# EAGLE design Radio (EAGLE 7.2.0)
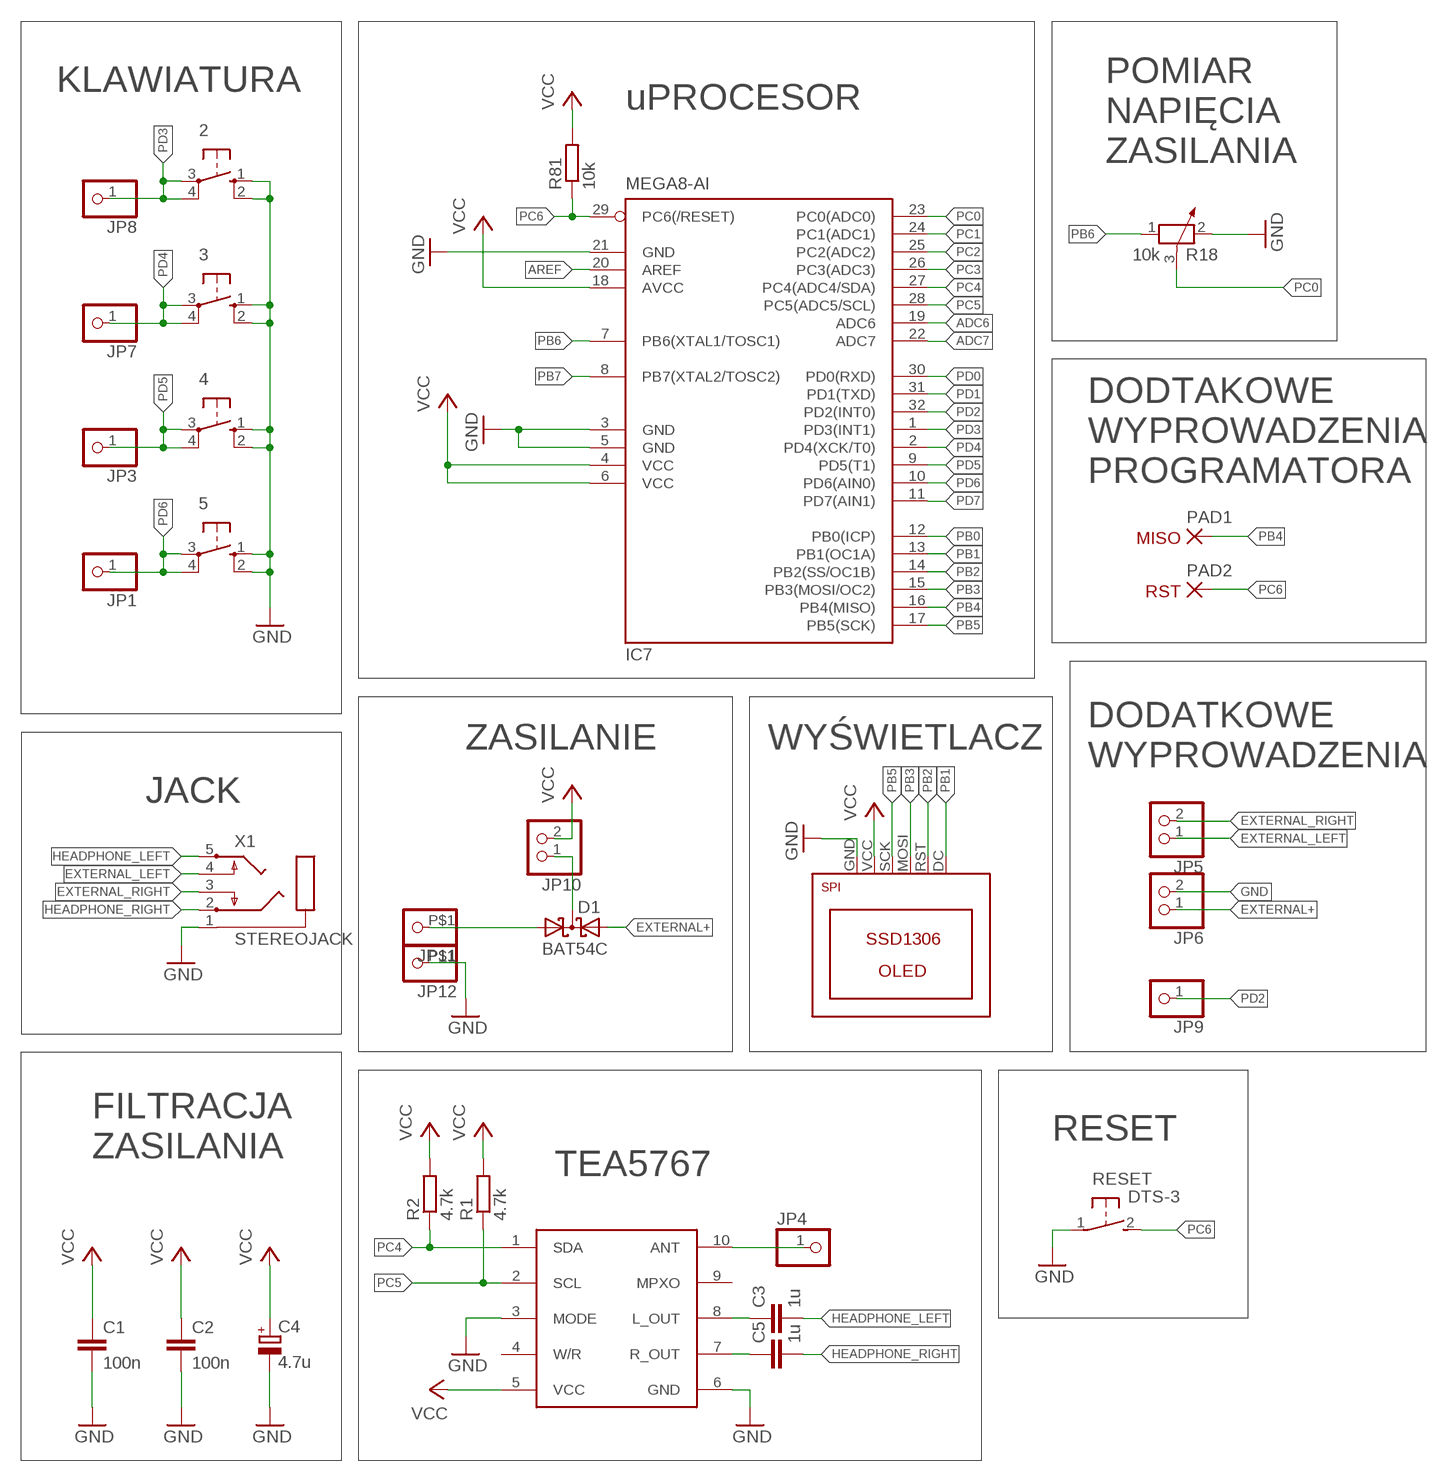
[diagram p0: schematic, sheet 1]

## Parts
2  10-XX  [B3F-10XX]
3  10-XX  [B3F-10XX]
4  10-XX  [B3F-10XX]
5  10-XX  [B3F-10XX]
C1  100n  C-EUC0805  [C0805]
C2  100n  C-EUC0805  [C0805]
C3  1u  C-EUC0805  [C0805]
C4  4.7u  CPOL-EUB/3528-21R  [B/3528-21R]
C5  1u  C-EUC0805  [C0805]
D1  BAT54C  [SOT23]
IC7  MEGA8-AI  [TQFP32-08]
JP1  PINHD-1X01_2.54-90°  [1X01/90]
JP3  PINHD-1X01_2.54-90°  [1X01/90]
JP4  PINHD-1X01_2.54-90°  [1X01/90]
JP5  PINHD-1X02_2.54  [1X02]
JP6  PINHD-1X02_2.54  [1X02]
JP7  PINHD-1X01_2.54-90°  [1X01/90]
JP8  PINHD-1X01_2.54-90°  [1X01/90]
JP9  PINHD-1X01_2.54-90°  [1X01/90]
JP10  PINHD-1X02_2.54  [1X02]
JP11  PINHD-1X01  [1X01_OFFSET]
JP12  PINHD-1X01  [1X01_OFFSET]
PAD1  SMD2  [SMD1,27-2,54]
PAD2  SMD2  [SMD1,27-2,54]
R1  4.7k  R-EU_R0805  [R0805]
R2  4.7k  R-EU_R0805  [R0805]
R18  10k  POTENTIOMETER_  [WH06-2A]
R81  10k  R-EU_R0805  [R0805]
RESET  DTS-3  [DTS-3]
U$1  TEA5767BREAKOUT  [TEA5767MM2]
U$2  SPINEW  [SSD1306_SPI_NO_CS_NO_HOLES]
X1  STEREOJACK  [STX3100]

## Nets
ADC6: IC7.19(ADC6)
ADC7: IC7.22(ADC7)
AREF: IC7.20(AREF)
BATTERY+: D1.1(A1) JP11.P$1
EXTERNAL+: D1.2(A2) JP6.1
EXTERNAL_LEFT: JP5.1 X1.4
EXTERNAL_RIGHT: JP5.2 X1.3
GND: 2.1(S) 2.2(S1) 3.1(S) 3.2(S1) 4.1(S) 4.2(S1) 5.1(S) 5.2(S1) C1.2 C2.2 C4.- IC7.3(GND) IC7.5(GND) IC7.21(GND) JP6.2 JP12.P$1 R18.2 RESET.1 U$1.3(MODE) U$1.6(GND) U$2.GND X1.1
HEADPHONE_LEFT: C3.2 X1.5
HEADPHONE_RIGHT: C5.2 X1.2
N$1: JP4.1 U$1.10(ANT)
N$2: D1.3(CC) JP10.1
N$3: C3.1 U$1.8(L_OUT)
N$4: C5.1 U$1.7(R_OUT)
PB0: IC7.12(PB0(ICP))
PB1: IC7.13(PB1(OC1A)) U$2.DC
PB2: IC7.14(PB2(SS/OC1B)) U$2.RST
PB3: IC7.15(PB3(MOSI/OC2)) U$2.MOSI
PB4: IC7.16(PB4(MISO)) PAD1.1(P)
PB5: IC7.17(PB5(SCK)) U$2.SCK
PB6: IC7.7(PB6(XTAL1/TOSC1)) R18.1
PB7: IC7.8(PB7(XTAL2/TOSC2))
PC0: IC7.23(PC0(ADC0)) R18.3
PC1: IC7.24(PC1(ADC1))
PC2: IC7.25(PC2(ADC2))
PC3: IC7.26(PC3(ADC3))
PC4: IC7.27(PC4(ADC4/SDA)) R2.1 U$1.1(SDA)
PC5: IC7.28(PC5(ADC5/SCL)) R1.1 U$1.2(SCL)
PC6: IC7.29(PC6(/RESET)) PAD2.1(P) R81.1 RESET.2
PD0: IC7.30(PD0(RXD))
PD1: IC7.31(PD1(TXD))
PD2: IC7.32(PD2(INT0)) JP9.1
PD3: 2.3(P) 2.4(P1) IC7.1(PD3(INT1)) JP8.1
PD4: 3.3(P) 3.4(P1) IC7.2(PD4(XCK/T0)) JP7.1
PD5: 4.3(P) 4.4(P1) IC7.9(PD5(T1)) JP3.1
PD6: 5.3(P) 5.4(P1) IC7.10(PD6(AIN0)) JP1.1
PD7: IC7.11(PD7(AIN1))
VCC: C1.1 C2.1 C4.+ IC7.4(VCC) IC7.6(VCC) IC7.18(AVCC) JP10.2 R1.2 R2.2 R81.2 U$1.5(VCC) U$2.VCC
Unconnected: U$1.4(W/R) U$1.9(MPXO)

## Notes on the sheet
- KLAWIATURA
- uPROCESOR
- POMIAR
  NAPIĘCIA
  ZASILANIA
- DODTAKOWE
  WYPROWADZENIA
  PROGRAMATORA
- MISO
- RST
- ZASILANIE | WYŚWIETLACZ
- DODATKOWE
  WYPROWADZENIA
- JACK
- RESET
- FILTRACJA
  ZASILANIA
- TEA5767

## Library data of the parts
2-5 = switch-omron:10-XX: OMRON SWITCH; MPN: B3F-1000; OC_FARNELL: 176432; OC_NEWARK: 36M3542
C1-C3 C5 = rcl:C-EU: CAPACITOR, European symbol
C4 = rcl:CPOL-EU: POLARIZED CAPACITOR, European symbol
D1 = diode:BAT54C: Schottky Diodes Source: Fairchild .. BAT54.pdf
IC7 = atmel:MEGA8: MICROCONTROLLER 8 Kbytes FLASH, 1 kbytes SRAM, 512 bytes EEPROM, USART, 6-channel 10 bit ADC, 2-channel 8 bit ADC Pin compatible with Atmega48, ATMega88, ATMega168 Source: avr.lbr; MPN: ATMEGA8-16AU; OC_FARNELL: 9171371; OC_NEWARK: 73M8863
JP1 JP3 JP4 JP7-JP9 = pinhead_my:PINHD-1X01: PIN HEADER
JP5 JP6 JP10 = pinhead_my:PINHD-1X02: PIN HEADER
JP11 JP12 = pinhead-2:PINHD-1X01: PIN HEADER
PAD1 PAD2 = wirepad:SMD2: SMD PAD
R1 R2 R81 = rcl:R-EU_: RESISTOR, European symbol
R18 = potencjometr:POTENTIOMETER_: Potentiometer
RESET = switch-tact:DTS-3
U$1 = MyParts:TEA5767BREAKOUT
U$2 = ssd1306_breakout_board:SPI
X1 = adafruit:STEREOJACK: MIC/HEADPHONE JACK Stereo jack with two switches. Kycon STX3100, CUI SJ1-3555NG and/or 4UCon 05544

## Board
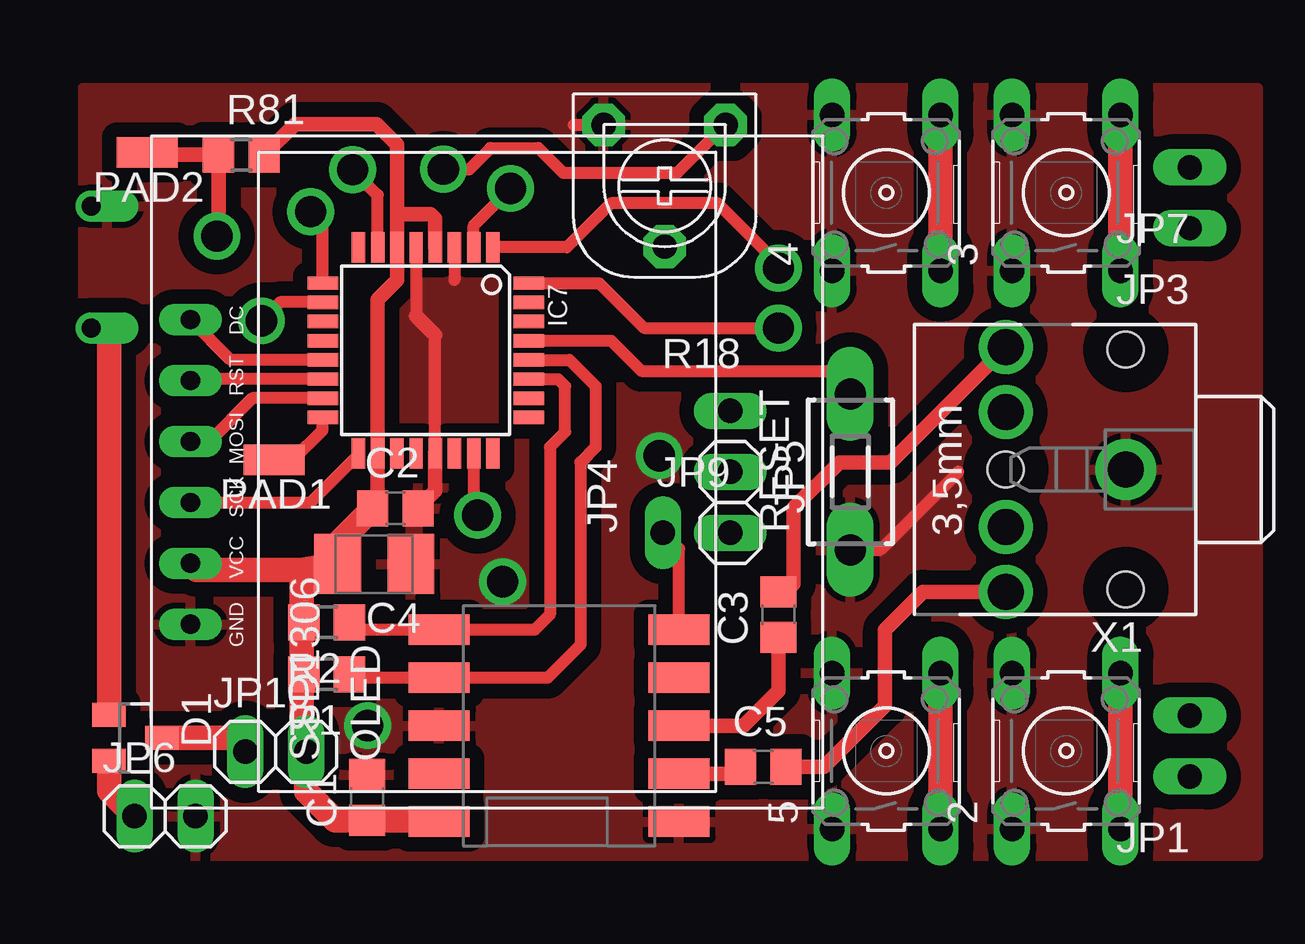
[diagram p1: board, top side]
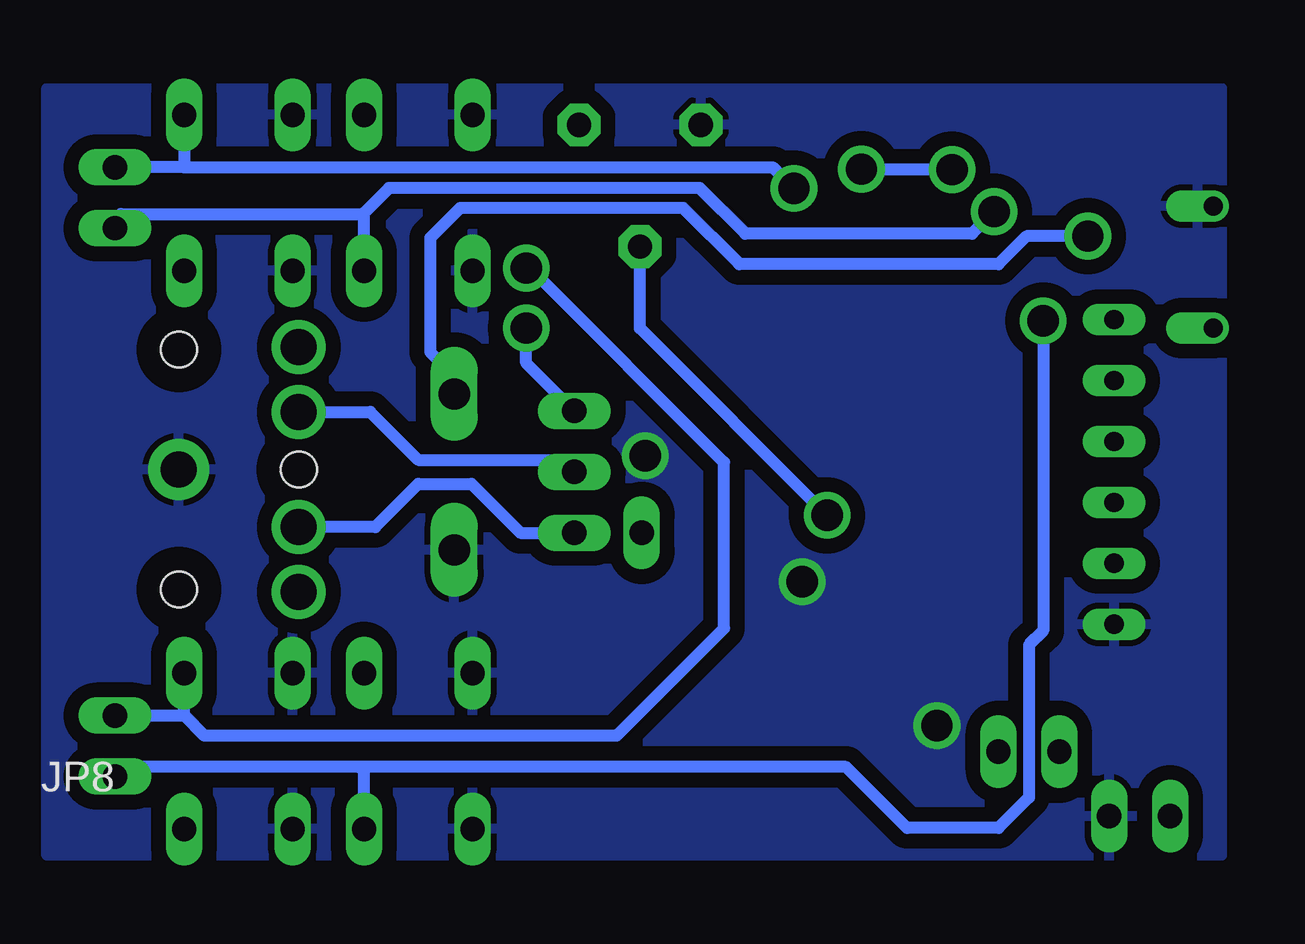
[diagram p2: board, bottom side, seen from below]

No outline drawn. Coordinates in mm, seen from the top.
Copper layers (1*16): Top 0.035mm / dielectric 1.5mm / Bottom 0.035mm
Design rules "default": minimum track width 10mil, minimum drill 24mil, track to track 8mil, track to pad 8mil, pad to pad 8mil, via to via 8mil, smd to smd 8mil, copper to edge 40mil, drill to drill 8mil, minimum pad ring 10mil, minimum via ring 8mil, stop-mask expansion 4mil, vias tented up to drill 0mil, thermal gap 10mil

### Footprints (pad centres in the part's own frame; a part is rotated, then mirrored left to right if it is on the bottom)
B3F-10XX = drill 1.016 long: 1 -3.251,2.261; 2 3.251,2.261; 3 -3.251,-2.261; 4 3.251,-2.261
C0805 = smd 1.3 x 1.5: 1 -0.95,0; 2 0.95,0
B/3528-21R = smd 1.95 x 2.5: + 1.525,0; - -1.525,0
SOT23 = smd 1 x 1.4: 1 -0.95,-1.1; 2 0.95,-1.1; 3 0,1.1
TQFP32-08 = smd 1.27 x 0.559: 1 -4.293,2.8; 2 -4.293,2; 3 -4.293,1.2; 4 -4.293,0.4; 5 -4.293,-0.4; 6 -4.293,-1.2; 7 -4.293,-2; 8 -4.293,-2.8; 17 4.293,-2.8; 18 4.293,-2; 19 4.293,-1.2; 20 4.293,-0.4; 21 4.293,0.4; 22 4.293,1.2; 23 4.293,2; 24 4.293,2.8 | smd 0.559 x 1.27: 9 -2.8,-4.293; 10 -2,-4.293; 11 -1.2,-4.293; 12 -0.4,-4.293; 13 0.4,-4.293; 14 1.2,-4.293; 15 2,-4.293; 16 2.8,-4.293; 25 2.8,4.293; 26 2,4.293; 27 1.2,4.293; 28 0.4,4.293; 29 -0.4,4.293; 30 -1.2,4.293; 31 -2,4.293; 32 -2.8,4.293
1X01/90 = drill 1.016 long: 1 0,0
1X02 = drill 1.016 long: 1 -1.27,0; 2 1.27,0
1X01_OFFSET = drill 0.8 offset: P$1 0,0
SMD1,27-2,54 = smd 1.27 x 2.54: 1 0,0
R0805 = smd 1.3 x 1.5: 1 -0.95,0; 2 0.95,0
WH06-2A = drill 1.016 pad 1.778 octagon: 1 -2.54,-2.54; 2 2.54,-2.54; 3 0,2.54
DTS-3 = drill 1.3 long: 1 -3.25,0; 2 3.25,0
TEA5767MM2 = smd 2.54 x 1.27: 1 -5,4; 2 -5,2; 3 -5,0; 4 -5,-2; 5 -5,-4; 6 5,-4; 7 5,-2; 8 5,0; 9 5,2; 10 5,4
SSD1306_SPI_NO_CS_NO_HOLES = drill 0.8 long: DC 6.35,12.37; GND -6.35,12.37; MOSI 1.27,12.37; RST 3.81,12.37; SCK -1.27,12.37; VCC -3.81,12.37
STX3100 = drill 1.5 pad 2.54: 1 2.7,-0.1 | drill 1.5: 2 7.7,5; 3 7.7,2.3; 4 7.7,-2.5; 5 7.7,-5.2 | hole 1.5: 2.7,4.9; 2.7,-5.1; 7.7,-0.1

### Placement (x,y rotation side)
2  52,13.37 90 top
3  52,36.63 90 top
4  44.5,36.63 90 top
5  44.5,13.37 90 top
C1  22.86,11.43 90 top
C2  24.04,23.48 0 top
C3  40.01,19.05 90 top
C4  23.16,21.16 180 top
C5  39.37,12.7 0 top
D1  13.2,13.91 270 top
IC7  25.3,30.07 270 top
JP1  57.15,12.3 90 top
JP3  57.15,35.16 90 top
JP4  35.19,22.46 0 top
JP5  38,23.73 270 top
JP6  14.44,10.64 0 top
JP7  57.15,37.7 90 top
JP8  57.15,14.84 90 bottom
JP9  38,27.54 90 top
JP10  19.05,13.34 0 top
JP11  11.37,31 0 top
JP12  11.37,36.08 0 top
PAD1  18.98,25.52 90 top
PAD2  13.69,38.31 90 top
R1  21.17,16.57 180 top
R2  21.17,18.73 180 top
R18  35.26,36.93 180 top
R81  17.61,38.22 0 top
RESET  43,25 90 top
U$1  30.86,14.41 0 top
U$2  27.86,25 90 top
X1  57.18,25 180 top

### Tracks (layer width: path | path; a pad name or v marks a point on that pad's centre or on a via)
BATTERY+
  Top 1.016: D1.1 12.1,30.48 12.1,31 JP11.P$1
EXTERNAL+
  Top 1.016: JP6.1 12.1,11.71 D1.2
EXTERNAL_LEFT
  Bottom 0.508: X1.4 46.5,27.5 44.5,25.5 38.5,25.5 JP5.1
EXTERNAL_RIGHT
  Bottom 0.508: X1.3 46.3,22.7 44.5,24.5 42.28,24.5 40.24,22.46 JP5.2
GND  (via drill 1.3 pad 1.78)
  Top 0.508: RESET.1 44.25,21.75 47.5,25 | 54.38,25 X1.1 | 32.5,39.25 R18.2 31.47,39.47 | IC7.21 25.7,30.7 | IC7.3 26.5,33 | IC7.5 24.9,31.5
  Top 0.61: C2.2 25.7,24.2 IC7.21 | 24.9,31.5 25.7,30.7
  other vias: 35.04,25.68 28.5,20.42 22.88,14.42
  pour Bottom (isolate 0.61): 11,9 60,9 60,41 11,41
  pour Top (isolate 0.61): 11,9 60,9 60,41 11,41
HEADPHONE_LEFT
  Top 0.61: X1.5 44.68,25.4 42.55,25.4 40.64,23.5 40.64,20.32 40.32,20 C3.2
HEADPHONE_RIGHT
  Top 0.61: X1.2 46.03,20 44.45,18.41 44.45,15.24 41.91,12.7 C5.2
N$1
  Top 0.508: U$1.10 35.86,21.79 JP4.1
N$2
  Top 1.016: JP10.1 17.2,13.91 D1.3
N$3
  Top 0.61: C3.1 40.01,15.88 38.55,14.41 U$1.8
N$4
  Top 0.61: U$1.7 38.42,12.41 C5.1
PB1
  Top 0.508: IC7.13 17.18,29.67 U$2.DC
PB2
  Top 0.508: IC7.14 15.55,28.87 U$2.RST
PB3
  Top 0.508: IC7.15 18.07,28.07 16.27,26.27 U$2.MOSI
PB4
  Top 0.508: IC7.16 21,26.73 19.79,25.52 PAD1.1
PB5
  Top 0.508: U$2.SCK 20.5,23.73 22.5,25.73 IC7.17
PB6  (via drill 1.3 pad 1.78)
  Top 0.508: R18.1 35.8,37.47 31.04,37.47 30,38.5 28,38.5 27.12,37.62 v26.04,37.62 | IC7.7 23.3,36.55 v22.25,37.59
  Bottom 0.508: v22.25,37.59 25.76,37.59 v26.04,37.62
PC0  (via drill 1.3 pad 1.78)
  Top 0.508: IC7.23 27.3,23.35 v27.46,23.19
  Bottom 0.508: v27.46,23.19 35.26,30.99 R18.3
PC4
  Top 0.508: IC7.27 30.82,28.87 31.11,28.57 31.11,26.67 30.48,26.04 30.48,19.05 29.84,18.41 U$1.1 22.43,18.41 R2.1
PC5
  Top 0.508: IC7.28 31.29,29.67 32.38,28.57 32.38,26.04 31.75,25.4 31.75,17.78 30.39,16.41 U$1.2 22.27,16.41 R1.1
PC6  (via drill 1.3 pad 1.78)
  Top 0.508: RESET.2 42.04,29.21 34.29,29.21 33.03,30.47 IC7.29
  Top 0.61: PAD2.1 13.79,38.22 R81.1 16.66,34.9 v16.59,34.83
  Bottom 0.508: RESET.2 43,29 44,30 44,34.75 42.75,36 33.46,36 31.11,33.66 20.32,33.66 19.15,34.83 v16.59,34.83
PD2  (via drill 1.3 pad 1.78)
  Top 0.508: IC7.32 32.53,32.87 34.41,31 v40,31
  Bottom 0.508: JP9.1 40,29.54 v40,31
PD3  (via drill 1.3 pad 1.78)
  Top 0.508: v40,33.5 40,33.66 37.47,36.2 33.02,36.2 31.19,34.36 IC7.1
  Top 0.61: 54.26,14.84 54.26,13.97
  Top 1.016: 2.3 54.26,13.97 2.4
  Bottom 0.508: 56.5,15 58,15 57.84,14.84 JP8.1 54.26,14.84 | 54.26,14.84 2.4 | 54.26,14.84 53.42,14 36.23,14 31.75,18.48 31.75,25.4 39.85,33.5 v40,33.5
PD4  (via drill 1.3 pad 1.78)
  Top 0.508: 54.26,37.7 54.26,37.5 | IC7.2 27.3,35.27 v28.84,36.81
  Top 0.61: 54.26,35.16 54.26,34.29
  Top 1.016: 3.4 54.26,37.5 54.26,34.29 3.3
  Bottom 0.508: 54.26,37.7 JP7.1 | 3.4 54.26,37.7 | 54.26,37.7 29.73,37.7 v28.84,36.81
PD5  (via drill 1.3 pad 1.78)
  Top 0.508: IC7.9 21.01,35.34 v20.5,35.84
  Top 1.016: 4.4 4.3
  Bottom 0.508: JP3.1 57.15,35.5 56.9,35.75 46.8,35.75 46.76,35.79 | v20.5,35.84 21.42,34.92 30.86,34.92 32.77,36.83 45.72,36.83 46.02,36.52 46.76,35.79 | 4.3 46.76,35.79
PD6  (via drill 1.3 pad 1.78)
  Top 0.508: IC7.10 19.23,32.07 v18.45,31.3
  Top 1.016: 5.3 5.4
  Bottom 0.508: 46.76,12.7 46.99,12.7 56.75,12.7 | 5.3 46.76,12.7 | v18.45,31.3 18.45,18.38 19.05,17.78 19.05,11.43 20.32,10.16 24.13,10.16 26.67,12.7 46.76,12.7
  Bottom 0.61: JP1.1 56.75,12.7
VCC
  Top 0.508: R1.2 20.22,17.68 | 20.22,17.68 20.12,17.78 | R2.2 20.22,17.88 20.32,17.78 20.22,17.68
  Top 0.61: C2.1 23.3,23.7 IC7.18 23.3,32.19 24.1,32.99 IC7.6 24.1,35.75 | IC7.4 25.7,35.55 25.5,35.75 24.1,35.75 | 24.1,35.75 24.1,38.65 23.25,39.5 19.85,39.5 R81.2
  Top 1.016: U$1.5 25.86,10.48 C1.1 21.52,10.48 20.32,11.68 JP10.2 20.32,13.02 20.12,13.21 20.12,17.78 20.12,20.92 | 20.12,20.92 15.77,20.92 U$2.VCC | 20.12,20.92 C4.+ 21.63,22.02 C2.1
